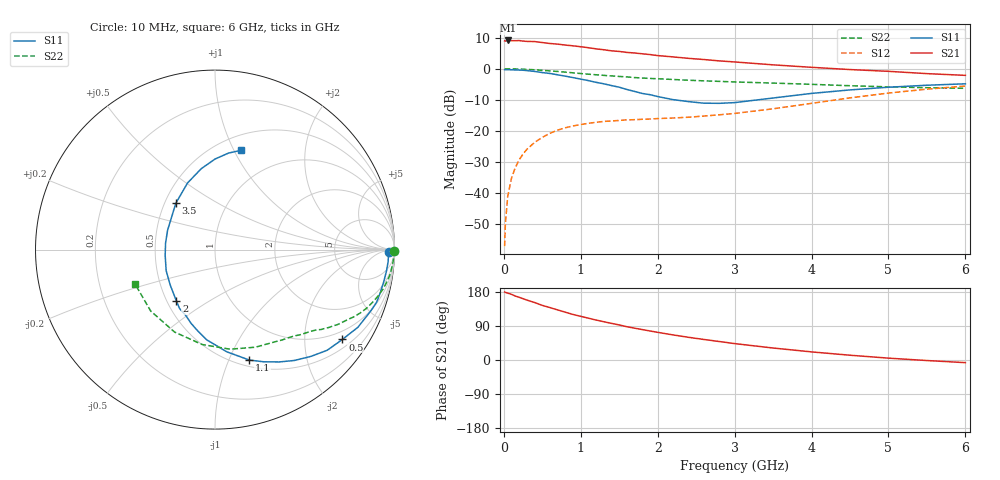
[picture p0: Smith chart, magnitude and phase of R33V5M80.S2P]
! SIEMENS Small Signal Semiconductors
! BFR181
! Si NPN RF Bipolar Junction Transistor in SOT23
! VCE = 3.5 V  IC = 0.8 mA
! Common Emitter S-Parameters:  May  1996
# GHz  S  MA  R  50
!  f  S11  S21  S12  S22
! GHz  MAG  ANG  MAG  ANG  MAG  ANG  MAG  ANG
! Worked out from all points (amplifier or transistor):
!   36 points, 10 MHz to 6 GHz, reference 50 ohm
!   highest |S21| = 9.1 dB at 50 MHz (marker M1)
!   |S21| within 3 dB of that: start of sweep to 1.302 GHz
!   unconditionally stable (mu >= 1): 2.134 GHz to 3.739 GHz
!   at 250 MHz: K = 0.14, MSG = 18.2 dB, |S12| = -27.4 dB
!   at 1.4 GHz: K = 0.71, MSG = 11.3 dB, |S12| = -16.8 dB
!   at 6 GHz: K = 0.89, MSG = 1.7 dB, |S12| = -5.6 dB
!   S11 on the Smith chart (normalised r, x): 10 MHz: 54, -24; 500 MHz: 0.73, -2.99; 1.1 GHz: 0.57, -1.19; 2 GHz: 0.56, -0.37; 3.5 GHz: 0.57, +0.33; 6 GHz: 0.65, +1.07
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0.01  0.9695 -0.8  2.809 179.5  0.0014 96.3  0.9998 -0.3
0.02  0.9667 -1.5  2.789 178.4  0.0032 88.2  0.9949 -0.7
0.05  0.967 -3.9  2.853 176.5  0.0088 88.6  0.9971 -1.7
0.1  0.9628 -7.2  2.833 173.3  0.0175 86.2  0.9952 -3.4
0.15  0.9571 -10.7  2.828 168.7  0.0258 82.5  0.9918 -5.1
0.2  0.9521 -14.2  2.841 165.4  0.0344 80.7  0.9881 -6.7
0.3  0.9333 -21.4  2.755 158.1  0.0507 76.0  0.9768 -10.0
0.4  0.9063 -28.5  2.738 151.7  0.0654 71.6  0.9628 -13.1
0.5  0.8686 -35.2  2.638 144.1  0.0788 67.1  0.9432 -16.1
0.7  0.7995 -48.1  2.489 132.1  0.1029 59.7  0.9044 -21.3
0.8  0.7597 -54.4  2.404 126.1  0.1124 56.4  0.8826 -23.6
0.9  0.7206 -60.3  2.338 120.1  0.1204 53.5  0.8597 -25.8
1.1  0.6447 -72.7  2.179 110.3  0.1327 48.6  0.8182 -29.6
1.3  0.5728 -83.5  2.021 101.0  0.1423 44.9  0.7831 -32.9
1.6  0.4642 -101.8  1.83 87.8  0.1507 41.4  0.7397 -37.0
2  0.3571 -127.1  1.63 73.0  0.1581 41.0  0.6905 -42.0
2.2  0.3188 -141.4  1.551 66.2  0.1614 41.6  0.6724 -44.8
2.8  0.2779 172.3  1.339 48.8  0.1817 46.3  0.6271 -53.4
3.5  0.3385 130.1  1.156 31.6  0.227 50.6  0.5886 -67.5
4.5  0.457 99.7  0.971 12.6  0.34 48.1  0.5336 -97.7
5.5  0.5432 82.0  0.835 -1.4  0.4697 35.7  0.4955 -136.3
6  0.5729 75.1  0.783 -7.0  0.5275 27.5  0.4847 -156.5
